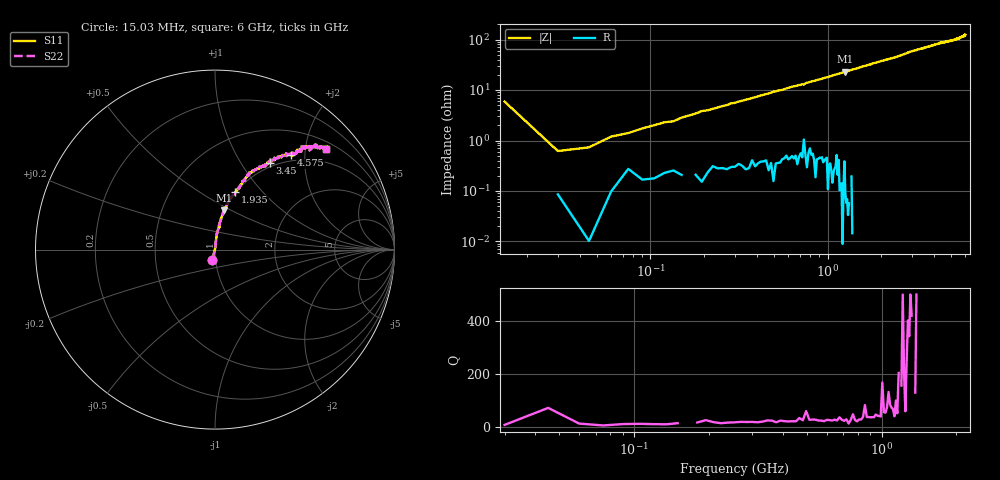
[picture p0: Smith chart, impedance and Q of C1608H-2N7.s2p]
!	Network	Analyzer	HP8753E.07.74:	Oct	30	2002	Serial	No.	JP38451487
!	Hewlett-Packard
!	7	Sep	2009	10:10:29
!	Frequency	S11	S21	S12	S22
#	HZ	S	RI	R	50
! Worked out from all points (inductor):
!   400 points, 15.03 MHz to 6 GHz, reference 50 ohm
!   read as one part in series: L = 2.92 nH near 45.03 MHz
!   highest Q = 342 at 1.26 GHz (marker M1), where L = 2.9 nH
!   S11 on the Smith chart (normalised r, x): 15.03 MHz: 0.96, -0.11; 1.935 GHz: 0.99, +0.72; 3.45 GHz: 0.93, +1.35; 4.575 GHz: 0.89, +1.73; 6 GHz: 0.65, +2.44
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1.502992e7  -0.0152 -0.0574  1.02 0.0574  1.02 0.0574  -0.0152 -0.0574
3.002985e7  0.000791 0.00612  0.999 -0.00612  0.999 -0.00612  0.000791 0.00612
4.502978e7  0.000312 0.00732  1 -0.00732  1 -0.00732  0.000312 0.00732
6.00297e7  0.00124 0.0119  0.999 -0.0119  0.999 -0.0119  0.00124 0.0119
1.200294e8  0.00259 0.0227  0.997 -0.0227  0.997 -0.0227  0.00259 0.0227
1.95029e8  0.00296 0.0381  0.997 -0.0381  0.997 -0.0381  0.00296 0.0381
2.850286e8  0.00577 0.0538  0.994 -0.0538  0.994 -0.0538  0.00577 0.0538
4.950275e8  0.0102 0.0919  0.99 -0.0919  0.99 -0.0919  0.0102 0.0919
1.020025e9  0.0356 0.177  0.964 -0.177  0.964 -0.177  0.0356 0.177
1.260024e9  0.051 0.218  0.949 -0.218  0.949 -0.218  0.051 0.218
1.93502e9  0.114 0.322  0.886 -0.322  0.886 -0.322  0.114 0.322
2.01002e9  0.121 0.329  0.879 -0.329  0.879 -0.329  0.121 0.329
3.015015e9  0.247 0.462  0.753 -0.462  0.753 -0.462  0.247 0.462
3.450013e9  0.304 0.485  0.696 -0.485  0.696 -0.485  0.304 0.485
4.00501e9  0.375 0.527  0.625 -0.527  0.625 -0.527  0.375 0.527
4.575007e9  0.425 0.526  0.575 -0.526  0.575 -0.526  0.425 0.526
5.010005e9  0.472 0.554  0.528 -0.554  0.528 -0.554  0.472 0.554
5.535002e9  0.527 0.553  0.473 -0.553  0.473 -0.553  0.527 0.553
5.565002e9  0.56 0.586  0.44 -0.586  0.44 -0.586  0.56 0.586
5.595002e9  0.537 0.572  0.463 -0.572  0.463 -0.572  0.537 0.572
5.625002e9  0.569 0.577  0.431 -0.577  0.431 -0.577  0.569 0.577
6e9  0.62 0.563  0.38 -0.563  0.38 -0.563  0.62 0.563
